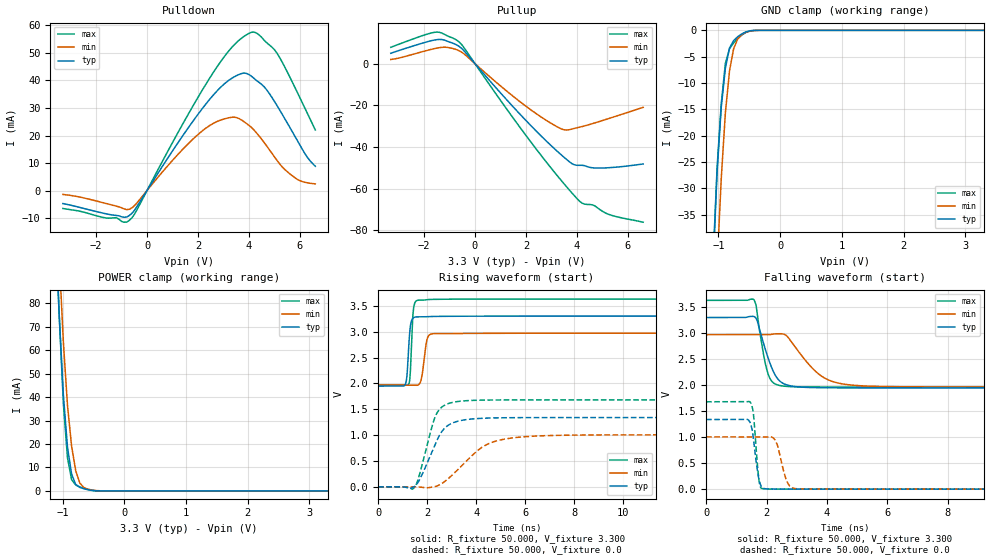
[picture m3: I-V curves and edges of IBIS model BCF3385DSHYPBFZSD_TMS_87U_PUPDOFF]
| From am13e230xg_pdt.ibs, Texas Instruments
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|   Model BCF3385DSHYPBFZSD_TMS_87U_PUPDOFF
[Model] BCF3385DSHYPBFZSD_TMS_87U_PUPDOFF
Model_type I/O
Polarity   Non-Inverting
Enable   Active-Low
Vinl =  0.990V
Vinh =  2.310V
Vmeas =  1.650V
C_comp   0.559pF   0.509pF   0.619pF
[Model Spec]
Vinh   2.310V   2.079V   2.541V
Vinl   0.990V   0.891V   1.089V
Vmeas   1.650V   1.485V   1.815V
[Temperature Range]   25.000   0.155k   -40.000
[Voltage Range]   3.300V   2.970V   3.630V
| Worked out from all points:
|   slope of the pulldown table from 0 to 0.495 V, typ, clamps not added: 68.5 ohm
|   slope of the pullup table from 0 to 0.495 V, typ, clamps not added: 70.6 ohm
|   GND clamp passes 1 mA (typ) near -0.66 V on its own axis
|   POWER clamp passes 1 mA (typ) near -0.66 V on its own axis
|   rising waveform, R_fixture 50.000, V_fixture 3.300: 20-80 % time 110ps typ, 163ps min, 90.4ps max; typ from 1.95 V to 3.3 V
|   rising waveform, R_fixture 50.000, V_fixture 0.0: 20-80 % time 779ps typ, 1.42ns min, 574ps max; typ from 0 V to 1.34 V
|   falling waveform, R_fixture 50.000, V_fixture 3.300: 20-80 % time 474ps typ, 934ps min, 300ps max; typ from 3.3 V to 1.95 V
|   falling waveform, R_fixture 50.000, V_fixture 0.0: 20-80 % time 179ps typ, 262ps min, 135ps max; typ from 1.34 V to 0 V
[Pulldown]
|Voltage   I(typ)   I(min)   I(max)
-3.3V     -4.742mA   -1.441mA   -6.54mA
-700mV    -9.13mA    -6.846mA   -10.89mA
-400mV    -5.894mA   -4.558mA   -7.098mA
1.4V      19.9mA     14.97mA    24.17mA
2.4V      32.5mA     23.27mA    40.01mA
3.4V      41.22mA    26.67mA    52.78mA
3.8V      42.69mA    25.06mA    56.01mA
4.1V      41.53mA    22.89mA    57.54mA
4.6V      37.66mA    17.36mA    54.59mA
5.1V      30.85mA    10.91mA    49.89mA
5.9V      18.1mA     4.028mA    35.58mA
6.6V      8.814mA    2.416mA    22.04mA
[Pullup]
|Voltage   I(typ)   I(min)   I(max)
-3.3V     4.951mA    1.968mA    7.808mA
-1.5V     11.48mA    7.414mA    15.11mA
-700mV    8.857mA    6.582mA    11.1mA
-400mV    5.719mA    4.386mA    7.142mA
2V        -27.27mA   -20.43mA   -34.44mA
3.5V      -44.98mA   -31.75mA   -57.71mA
3.9V      -48.52mA   -31.06mA   -63.34mA
4.2V      -48.76mA   -30.19mA   -66.89mA
4.6V      -49.94mA   -28.82mA   -67.71mA
4.9V      -50.09mA   -27.69mA   -69.99mA
5.4V      -49.79mA   -25.74mA   -72.9mA
6.6V      -48.13mA   -20.97mA   -76.04mA
[GND_clamp]
|Voltage   I(typ)   I(min)   I(max)
-3.3V     -1.006A    -883.6mA   -1.273A
-1.089V   -45.2mA    -63.83mA   -44.22mA
-1.022V   -26.88mA   -44.72mA   -26.06mA
-955mV    -14.62mA   -28.27mA   -14.02mA
-888mV    -7.183mA   -15.73mA   -6.291mA
-821mV    -3.37mA    -7.718mA   -3.478mA
-754mV    -1.948mA   -3.475mA   -2.39mA
-687mV    -1.208mA   -1.613mA   -1.554mA
-620mV    -663.5uA   -801.3uA   -867.2uA
-553mV    -281.3uA   -375.3uA   -374.8uA
-352mV    -1.803uA   -10.08uA   -2.106uA
3.3V      0A         0A         0A
[POWER_clamp]
|Voltage   I(typ)   I(min)   I(max)
-3.3V     1.772A     2.005A     1.902A
-1.122V   114.9mA    143mA      120.1mA
-1.055V   74.57mA    99.89mA    75.01mA
-988mV    40.96mA    63.5mA     37.28mA
-921mV    18.59mA    36.47mA    14.09mA
-854mV    7.17mA     19mA       4.772mA
-787mV    2.703mA    8.539mA    2.533mA
-720mV    1.495mA    3.291mA    1.714mA
-653mV    916.7uA    1.391mA    1.057mA
-586mV    491.6uA    704.5uA    530.7uA
-385mV    11.77uA    47.43uA    7.131uA
3.3V      0A         0A         0A
[Ramp]
| variable   typ   min   max
dV/dt_r   0.803/0.779n   0.603/1.418n   1.008/0.574n
dV/dt_f   0.812/0.474n   0.602/0.934n   1.000/0.300n
R_load = 50.000
[Rising Waveform]
R_fixture= 50.000
V_fixture= 3.300
V_fixture_min= 2.970
V_fixture_max= 3.630
|time   V(typ)   V(min)   V(max)
0s        1.947V     1.966V     1.964V
1.089ns   1.963V     1.966V     1.965V
1.174ns   2.154V     1.966V     1.963V
1.25ns    2.736V     1.966V     1.986V
1.309ns   3.092V     1.966V     2.19V
1.432ns   3.267V     1.965V     3.41V
1.63ns    3.286V     1.97V      3.608V
1.998ns   3.289V     2.859V     3.619V
2.246ns   3.294V     2.96V      3.624V
25ns      3.3V       2.97V      3.63V
[Rising Waveform]
R_fixture= 50.000
V_fixture= 0.0
V_fixture_min= 0.0
V_fixture_max= 0.0
|time   V(typ)   V(min)   V(max)
0s        1.248uV    1.099uV    1.113uV
1.474ns   963.4uV    647.9uV    -16.94mV
1.665ns   117.8mV    -3.519mV   201.9mV
2.194ns   678.4mV    -6.423mV   1.163V
2.373ns   872.9mV    10.75mV    1.404V
2.728ns   1.141V     107.7mV    1.582V
3.226ns   1.265V     320.4mV    1.648V
4.455ns   1.329V     822.7mV    1.677V
6.105ns   1.338V     973mV      1.68V
25ns      1.339V     1.005V     1.68V
[Falling Waveform]
R_fixture= 50.000
V_fixture= 3.300
V_fixture_min= 2.970
V_fixture_max= 3.630
|time   V(typ)   V(min)   V(max)
0s        3.3V       2.97V      3.63V
1.579ns   3.32V      2.97V      3.643V
1.657ns   3.281V     2.97V      3.526V
1.867ns   2.872V     2.97V      2.699V
2.062ns   2.507V     2.97V      2.198V
2.304ns   2.177V     2.986V     2.018V
2.574ns   2.027V     2.98V      1.981V
3.796ns   1.95V      2.183V     1.964V
4.916ns   1.947V     1.996V     1.964V
25ns      1.947V     1.966V     1.964V
[Falling Waveform]
R_fixture= 50.000
V_fixture= 0.0
V_fixture_min= 0.0
V_fixture_max= 0.0
|time   V(typ)   V(min)   V(max)
0s        1.339V     1.005V     1.68V
1.474ns   1.257V     1.005V     1.662V
1.572ns   949.6mV    1.005V     1.421V
1.691ns   385.6mV    1.005V     515.2mV
1.758ns   167.9mV    1.005V     136.6mV
1.896ns   16.86mV    1.005V     7.503mV
2.28ns    1.832mV    945.7mV    1.454mV
2.695ns   731.9uV    125.9mV    409.2uV
3.023ns   346.7uV    6.842mV    137.9uV
25ns      18.51nV    163.2nV    42.26nV
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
